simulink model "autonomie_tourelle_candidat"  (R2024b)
settings: Solver=VariableStepAuto  StartTime=0.0  StopTime=2  RelTol=1e-3  AbsTol=1e-3
libraries: fl_lib x6, nesl_utility x6, batteryecm_lib x1, ee_lib x1, sdl_lib x1

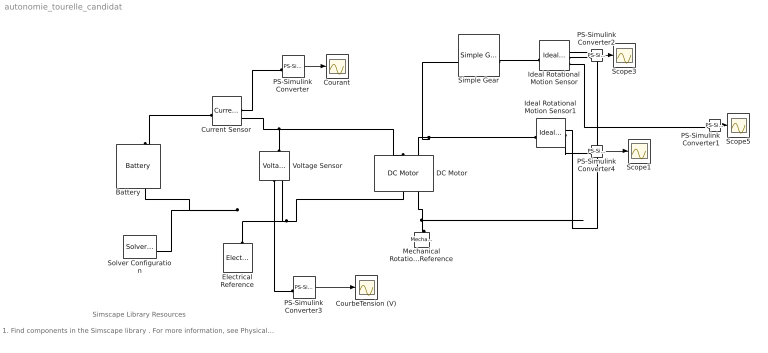
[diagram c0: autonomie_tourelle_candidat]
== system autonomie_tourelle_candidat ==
  note: 1. Find components in the Simscape library . For more information, see Physical Modeling - Blocks . 2. Connect the components to form a physical network. For more information, see Essential Steps for Constructing a Physical Model . 3. Explore simulation results using sscexplore
  note: Simscape Library Resources
  Battery : batteryecm_lib/Battery  Vnom=0 V  prm_dir=simscape.enum.battery.prm_dir.disabled  R1_dis=2 Ohm  R1_ch=2 Ohm  R1=0.06 Ohm  prm_AH=2  AH=0 hr*A  V1=0 V  AH1=0.3 hr*A  prm_R2=2  R2=inf Ohm  Tmeas=298.15 K  charge_measurement_port=simscape.enum.battery.enable.no  prm_dyn=simscape.enum.battery.prm_dyn.off  Rp1=0.005 Ohm  tau1=30 s  Rp2=0.005 Ohm  tau2=30 s  Rp3=0.005 Ohm  tau3=30 s  Rp4=0.005 Ohm  tau4=30 s  Rp5=0.005 Ohm  tau5=30 s  prm_fade=simscape.enum.battery.prm_fade.disabled  N_fade=100  AH_fade=45 A*hr  R1_fade=2.02 Ohm  R1_ch_fade=2.02 Ohm  V1_fade=10.35 V  prm_age=simscape.enum.battery.prm_age.disabled  prm_age_OCV=simscape.enum.battery.prm_age_OCV.OCV  OCV_age=0.9  SOC_age=60  Tmeas_age=298.15 K  delta_time_age_vec=[0] d  temperature_age_vec=[273] K  OCV_scaling_age=2.2134e6  OCV_offset_age=1.632e6  temp_exp_age=0.515833569 V  t_exp_age=0.75  Vnom_T2=12 V  R1_T2=2.2 Ohm  R1_T2_dis=2.2 Ohm  R1_T2_ch=2.2 Ohm  V1_T2=11.4 V  R2_T2=2200 Ohm  Rp1_T2=0.005 Ohm  tau1_T2=30 s  Rp2_T2=0.005 Ohm  tau2_T2=30 s  Rp3_T2=0.005 Ohm  tau3_T2=30 s  Rp4_T2=0.005 Ohm  tau4_T2=30 s  Rp5_T2=0.005 Ohm  tau5_T2=30 s  Tmeas2=273.15 K  thermal_port=simscape.enum.thermaleffects.omit  thermal_mass=30000 J/K  i_specify=off  i_priority=None  i=0 A  i_nominal_specify=off  i_nominal_value=1  i_nominal_unit=A  v_specify=off  v_priority=None  v=0 V  v_nominal_specify=off  v_nominal_value=1  v_nominal_unit=V  charge_specify=on  charge_priority=High  charge=0.75 hr*A  charge_nominal_specify=on  charge_nominal_value=0.75  charge_nominal_unit=A*hr  num_cycles_specify=off  num_cycles_priority=High  num_cycles=0  num_cycles_nominal_specify=off  num_cycles_nominal_value=1  num_cycles_nominal_unit=1  temperature_specify=off  temperature_priority=High  temperature=298.15 K  temperature_nominal_specify=off  temperature_nominal_value=1  temperature_nominal_unit=K
  Courant : Scope
  CourbeTension (V) : Scope
  Current Sensor : fl_lib/Electrical/Electrical Sensors/Current Sensor
  DC Motor : ee_lib/Electromechanical/Brushed Motors/DC Motor  field_option=ee.enum.field_option.pm  Rf=100 Ohm  Lf=1 H  Laf=0.15 H  If0=0 A  parameterization=1  Ra=0 Ohm  La=0 mH  emf_or_torque=1  Kv=0.0145 V/(rad/s)  Ki=6.876e-4 N*m/A  T_stall=0.24e-3 N*m  w_max=19100 rpm  w_rated=15000 rpm  P_rated=0.08 W  V_rated=1.5 V  lam_param=1  i_noload=0 A  V_i_noload=1.5 V  J=1 g*cm^2  lam=0 N*m/(rad/s)  speed0=0 rpm  t_fault_armature=1 s  t_fault_field=1 s  fault_action=simscape.enum.assert.action.none  alpha=3.93e-3 1/K  Tmeas=25 degC  thermal_mass=100 J/K  initial_temperature=25 degC
  Electrical Reference : fl_lib/Electrical/Electrical Elements/Electrical Reference
  Ideal Rotational Motion Sensor : fl_lib/Mechanical/Mechanical Sensors/Ideal Rotational Motion Sensor  reference=foundation.enum.MeasurementReference.difference  acceleration_port=false  velocity_port=true  position_port=true  wrap_angle=false  offset=0 rad
  Ideal Rotational Motion Sensor1 : fl_lib/Mechanical/Mechanical Sensors/Ideal Rotational Motion Sensor  reference=foundation.enum.MeasurementReference.difference  acceleration_port=false  velocity_port=true  position_port=true  wrap_angle=false  offset=0 rad
  Mechanical Rotational Reference : fl_lib/Mechanical/Rotational Elements/Mechanical Rotational Reference
  PS-Simulink Converter : nesl_utility/PS-Simulink Converter  PhysicalDomain=network_engine_domain  SubClassName=ps_output  LeftPortType=input  RightPortType=output  PseudoPeriodic=off  Frequencies=[]  VectorFormat=1-D array  Unit=A  AffineConversion=off
  PS-Simulink Converter1 : nesl_utility/PS-Simulink Converter  PhysicalDomain=network_engine_domain  SubClassName=ps_output  LeftPortType=input  RightPortType=output  PseudoPeriodic=off  Frequencies=[]  VectorFormat=1-D array  Unit=inherit  AffineConversion=off
  PS-Simulink Converter2 : nesl_utility/PS-Simulink Converter  PhysicalDomain=network_engine_domain  SubClassName=ps_output  LeftPortType=input  RightPortType=output  PseudoPeriodic=off  Frequencies=[]  VectorFormat=1-D array  Unit=rad/s  AffineConversion=off
  PS-Simulink Converter3 : nesl_utility/PS-Simulink Converter  PhysicalDomain=network_engine_domain  SubClassName=ps_output  LeftPortType=input  RightPortType=output  PseudoPeriodic=off  Frequencies=[]  VectorFormat=1-D array  Unit=1  AffineConversion=off
  PS-Simulink Converter4 : nesl_utility/PS-Simulink Converter  PhysicalDomain=network_engine_domain  SubClassName=ps_output  LeftPortType=input  RightPortType=output  PseudoPeriodic=off  Frequencies=[]  VectorFormat=1-D array  Unit=rad/s  AffineConversion=off
  Scope1 : Scope
  Scope3 : Scope
  Scope5 : Scope
  Simple Gear : sdl_lib/Gears/Simple Gear  ratio=368  rotation_direction=3-2*(1)  friction_model=sdl.enum.gear_efficiencies_load.off  T_noload=0.1 N*m  T_nom=5 N*m  efficiency_nom=0.8  efficiency=0.8  temperature_TLU=[280, 300, 320] K  load_TLU=[1, 5, 10] N*m  efficiency_TLU=[.95, .9, .85]  efficiency_TLU2=[.85, .8, .75; .95, .9, .85; .85, .8, .7]  w_thr=0.01 rad/s  pwr_thr=0.001 W  enable_backlash=false  hardstop_model=simscape.enum.hardstop.smooth  backlash_distance=1e-3 mm  r_base=0.1 m  transition=1e-4 mm  backlash_stiffness=1e6 N/m  backlash_damping=1e3 N*s/m  coeff_rest=0.7  v_tol=0.001 m/s  f_tol=0 N  mu_visc=[0.000000763, 0] N*m/(rad/s)  thermal_mass=50 J/K  temperature_specify=off  temperature_priority=High  temperature=300 K  temperature_nominal_specify=off  temperature_nominal_value=1  temperature_nominal_unit=K  x_backlash_specify=off  x_backlash_priority=None  x_backlash=0 mm  x_backlash_nominal_specify=off  x_backlash_nominal_value=1  x_backlash_nominal_unit=mm  f_hardstop_specify=off  f_hardstop_priority=None  f_hardstop=0 N  f_hardstop_nominal_specify=off  f_hardstop_nominal_value=1  f_hardstop_nominal_unit=N  v_backlash_specify=off  v_backlash_priority=None  v_backlash=0 m/s  v_backlash_nominal_specify=off  v_backlash_nominal_value=1  v_backlash_nominal_unit=m/s
  Solver Configuration : nesl_utility/Solver Configuration  PhysicalDomain=network_engine_domain  SubClassName=solver  LeftPortType=input  RightPortType=generic  Tones=[]  Harmonics=[]  SimulateNoise=off  Profile=off  UseLocalSampling=off  EnableSwitchedLinearOptims=on  FrequencyDomain=off  UseCCode=off  RelTol=0.001  AbsTol=1e-06  MinStep=1e-09  ToWorkspace=off  RevertToSquareIcSolve=off  NumHomotopyIterations=100  PhasorMode=off  PhasorModeNumHarmonics=1  ConsistencySolver=NEWTON_FTOL  IndexReductionMethod=DerivativeReplacement  DoDC=off  ResidualTolerance=1e-9  ConsistencyTolSource=GLOBAL  ConsistencyAbsTol=0.001  ConsistencyRelTol=0.001  ConsistencyTolFactor=0.001  UseLocalSolver=off  LocalSolverChoice=NE_BACKWARD_EULER_ADVANCER  ResolveIndetEquations=on  FunctionEvalNumThread=1  LocalSolverSampleTime=.001  DoFixedCost=off  MaxNonlinIter=3  MaxModeIter=2  ComputeImpulses=off  ImpulseIterations=2  LinearAlgebra=Sparse  LinearAlgebraNumThread=0  EquationFormulation=NE_TIME_EF  DelaysMemoryBudget=1024  AutomaticFiltering=on  FilteringTimeConstant=0.001  PartitionStorageMethod=AS_NEEDED  PartitionMemoryBudget=1024  PartitionMethod=FAST  MultibodyUseLocalSolver=off  MultibodyLocalSolverChoice=ODE1  MultibodyLocalSolverSampleTime=0.001
  Voltage Sensor : fl_lib/Electrical/Electrical Sensors/Voltage Sensor
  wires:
  PS-Simulink Converter2/1 -> Scope3/1
  PS-Simulink Converter4/1 -> Scope1/1
  PS-Simulink Converter1/1 -> Scope5/1
  PS-Simulink Converter/1 -> Courant/1
  PS-Simulink Converter3/1 -> CourbeTension (V)/1
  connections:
  Ideal Rotational Motion Sensor/RConn2 -- PS-Simulink Converter2/LConn1
  Voltage Sensor/LConn1 -- DC Motor/LConn1 -- Current Sensor/RConn2
  Mechanical Rotational Reference/LConn1 -- DC Motor/RConn2 -- Ideal Rotational Motion Sensor1/RConn1 -- Ideal Rotational Motion Sensor/RConn1
  Ideal Rotational Motion Sensor1/LConn1 -- DC Motor/LConn2 -- Simple Gear/LConn1
  Ideal Rotational Motion Sensor1/RConn2 -- PS-Simulink Converter4/LConn1
  Simple Gear/RConn1 -- Ideal Rotational Motion Sensor/LConn1
  Ideal Rotational Motion Sensor/RConn3 -- PS-Simulink Converter1/LConn1
  Electrical Reference/LConn1 -- DC Motor/RConn1 -- Voltage Sensor/RConn2 -- Battery/RConn1 -- Solver Configuration/RConn1
  Current Sensor/RConn1 -- PS-Simulink Converter/LConn1
  Voltage Sensor/RConn1 -- PS-Simulink Converter3/LConn1
  Current Sensor/LConn1 -- Battery/LConn1
